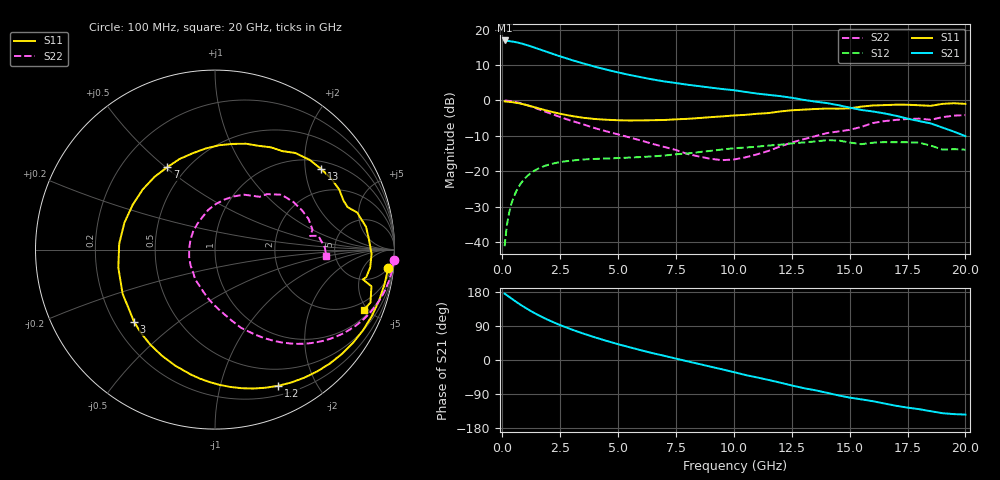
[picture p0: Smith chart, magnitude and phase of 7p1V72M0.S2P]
! Infineon Technologies  Discrete & RF Semiconductors
! bfp620
! VCE =  1.7 V,  IC =  2.0 mA
! Common Emitter S-Parameters:  Sep 2002
# GHz  S  MA  R  50
!  f  S11  S21  S12  S22
! GHz  MAG  ANG  MAG  ANG  MAG  ANG  MAG  ANG
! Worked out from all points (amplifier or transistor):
!   59 points, 100 MHz to 20 GHz, reference 50 ohm
!   highest |S21| = 16.9 dB at 100 MHz (marker M1)
!   |S21| within 3 dB of that: start of sweep to 1.831 GHz
!   unconditionally stable (mu >= 1): 5.794 GHz to 13.98 GHz; 14.01 GHz to 15.67 GHz; 17.56 GHz to end of sweep
!   at 1 GHz: K = 0.16, MSG = 18.8 dB, |S12| = -21.8 dB
!   at 5.5 GHz: K = 0.96, MSG = 11.7 dB, |S12| = -16.1 dB
!   at 20 GHz: K = 1.39, MAG = -1.8 dB, |S12| = -13.9 dB
!   S11 on the Smith chart (normalised r, x): 100 MHz: 5, -18; 1.2 GHz: 0.30, -1.52; 3 GHz: 0.28, -0.36; 7 GHz: 0.40, +0.51; 13 GHz: 1.21, +2.43; 20 GHz: 1.40, -4.75
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0.1  0.9709 -5.9  7.032 175.0  0.0088 83.9  0.998 -3.4
0.3  0.9573 -17.1  6.884 166.5  0.0265 80.8  0.9857 -10.0
0.5  0.9397 -28.4  6.726 157.8  0.0438 74.1  0.9628 -16.4
0.7  0.9157 -39.3  6.524 149.4  0.06 67.4  0.9314 -22.4
0.9  0.8862 -49.9  6.273 141.5  0.0745 60.9  0.8937 -28.1
1.2  0.8366 -65.1  5.848 130.4  0.0928 52.2  0.8308 -35.7
1.6  0.7698 -83.7  5.283 117.1  0.1112 42.2  0.746 -44.3
2  0.7095 -100.8  4.764 105.3  0.1241 33.9  0.669 -51.4
2.4  0.6608 -116.7  4.297 94.6  0.1332 27.2  0.601 -57.5
3  0.6044 -138.2  3.718 80.4  0.1421 18.7  0.5157 -65.5
3.5  0.5704 -154.5  3.331 69.7  0.1473 13.0  0.46 -71.5
4  0.548 -169.4  2.998 59.8  0.1498 8.1  0.407 -76.7
5  0.5265 163.4  2.49 41.7  0.1542 1.3  0.3327 -86.6
6  0.524 140.2  2.128 25.6  0.1594 -3.9  0.2716 -98.7
7  0.5307 120.1  1.858 11.0  0.1673 -7.9  0.2209 -112.7
9  0.5821 87.6  1.519 -17.7  0.1949 -18.0  0.1501 -163.7
10.5  0.6273 67.2  1.321 -39.6  0.2169 -29.1  0.1576 141.1
13  0.7423 37.3  1.023 -74.0  0.2557 -47.8  0.2835 79.4
13.5  0.7584 31.6  0.965 -79.7  0.2638 -52.6  0.3128 71.0
15  0.7754 17.8  0.794 -99.2  0.2557 -72.1  0.3853 49.8
17  0.8725 -1.6  0.609 -120.7  0.2576 -84.4  0.5317 24.4
20  0.8954 -22.0  0.314 -144.0  0.2019 -106.2  0.6216 -3.4
